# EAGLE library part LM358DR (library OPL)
General purpose LOW Voltage, Rail-to-Rail Output Amplifiers http://www.fairchildsemi.com/ds/LM/LMV358.pdf
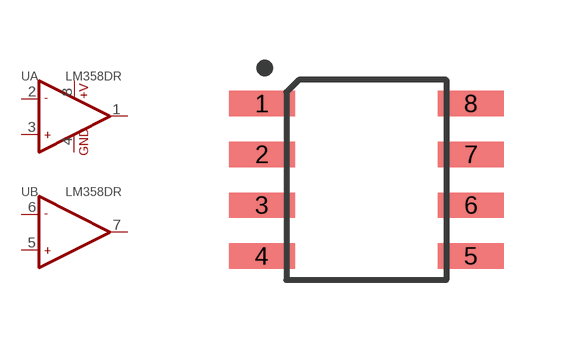
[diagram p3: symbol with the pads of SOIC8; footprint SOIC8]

Designator prefix U; gates A=OPAMP_2 B=OPAMP_2_1

## LM358DR-1110010P1  [SOIC8]
1  A:OUT1  out
2  A:-IN1  in
3  A:+IN1  in
4  A:GND  pwr
5  B:+IN2  in
6  B:-IN2  in
7  B:OUT2  out
8  A:+V  pwr

## Footprint SOIC8 (pad centres in mm)
Small Outline Package
smd 1.651 x 0.635: 1 -2.616,1.905; 2 -2.616,0.635; 3 -2.616,-0.635; 4 -2.616,-1.905; 5 2.616,-1.905; 6 2.616,-0.635; 7 2.616,0.635; 8 2.616,1.905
